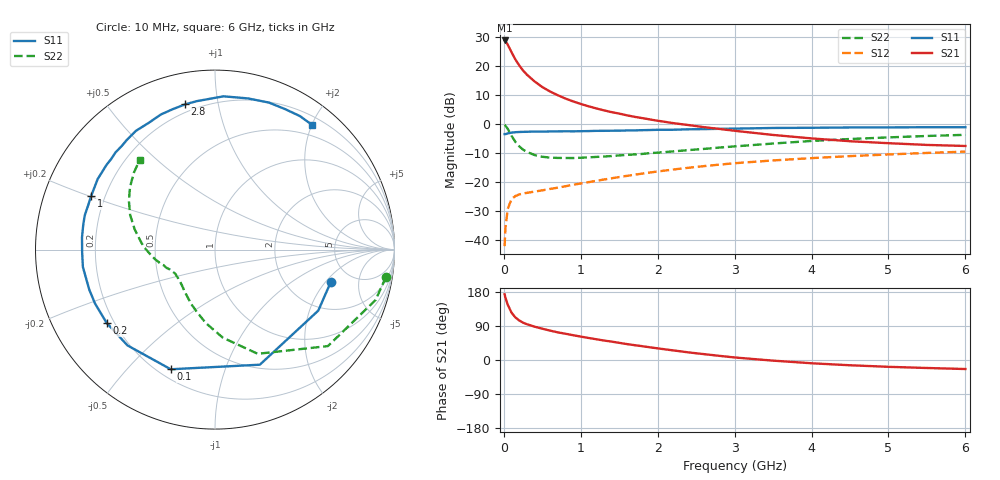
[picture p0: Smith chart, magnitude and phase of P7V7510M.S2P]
! SIEMENS Small Signal Semiconductors
! BFP196
! Si NPN RF Bipolar Junction Transistor in SOT143
! VCE = 0.75 V  IC = 10 mA
! Common Emitter S-Parameters:  May  1996
# GHz  S  MA  R  50
!  f  S11  S21  S12  S22
! GHz  MAG  ANG  MAG  ANG  MAG  ANG  MAG  ANG
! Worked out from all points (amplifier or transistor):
!   36 points, 10 MHz to 6 GHz, reference 50 ohm
!   highest |S21| = 28.8 dB at 10 MHz (marker M1)
!   |S21| within 3 dB of that: start of sweep to 79.95 MHz
!   unconditionally stable (mu >= 1): 837.1 MHz to end of sweep
!   at 250 MHz: K = 0.41, MSG = 21.2 dB, |S12| = -24.0 dB
!   at 1.4 GHz: K = 1.16, MAG = 9.0 dB, |S12| = -18.7 dB
!   at 6 GHz: K = 1.03, MAG = -0.1 dB, |S12| = -9.5 dB
!   S11 on the Smith chart (normalised r, x): 10 MHz: 3.45, -2.28; 100 MHz: 0.25, -0.67; 200 MHz: 0.17, -0.30; 1 GHz: 0.15, +0.20; 2.8 GHz: 0.16, +0.80; 6 GHz: 0.32, +2.00
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0.01  0.6697 -15.8  27.7 173.3  0.0078 83.1  0.9649 -9.1
0.02  0.6683 -30.6  26.84 164.9  0.0156 77.0  0.9378 -17.4
0.05  0.6882 -68.7  23.53 146.1  0.034 59.7  0.8276 -40.5
0.1  0.7109 -110.3  17.35 124.9  0.0508 42.8  0.6275 -67.7
0.15  0.723 -132.4  13.02 112.3  0.0572 34.6  0.4929 -84.9
0.2  0.7289 -146.0  10.3 104.3  0.0608 30.6  0.4125 -97.1
0.25  0.7328 -155.8  8.395 98.5  0.0634 29.1  0.3611 -106.4
0.3  0.7352 -162.3  7.102 94.4  0.0649 28.9  0.3304 -113.7
0.4  0.7424 -172.5  5.428 87.9  0.0683 29.0  0.2917 -124.7
0.5  0.7404 -179.0  4.346 82.6  0.0717 30.5  0.2722 -132.3
0.6  0.7442 174.7  3.647 77.6  0.0758 32.0  0.2637 -137.8
0.7  0.747 169.3  3.148 73.0  0.0797 33.8  0.2601 -142.1
0.8  0.7503 165.3  2.756 69.3  0.0843 34.8  0.2593 -145.6
1  0.752 156.6  2.219 61.8  0.0942 37.4  0.2616 -150.4
1.1  0.7557 152.7  2.026 58.2  0.0992 38.3  0.266 -152.3
1.6  0.7748 135.7  1.413 42.0  0.1275 39.9  0.2935 -161.1
2.2  0.7969 117.6  1.038 25.4  0.164 37.1  0.3369 -170.6
2.8  0.8262 101.6  0.824 11.0  0.1992 31.8  0.3924 178.5
3.5  0.8553 86.8  0.648 -1.7  0.2355 24.1  0.4606 166.0
4.5  0.8724 69.9  0.505 -13.9  0.2795 13.1  0.5518 150.4
5.5  0.8816 57.6  0.436 -21.1  0.3172 2.3  0.6221 136.7
6  0.8805 52.2  0.418 -23.8  0.3342 -3.7  0.6516 130.2
